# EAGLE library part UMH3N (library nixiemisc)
UMT6
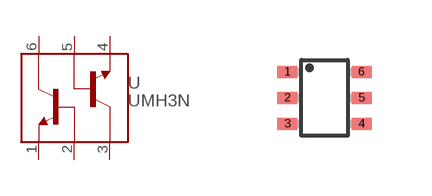
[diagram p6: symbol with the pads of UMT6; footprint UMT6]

Designator prefix U

## UMH3NUMT6  [UMT6]
1  E1  out
2  B1  in
3  C2  in
4  E2  out
5  B2  in
6  C1  in

## Footprint UMT6 (pad centres in mm)
UMT6 Package EIAJ: SC-88 Source: http://www.rohm.com/products/databook/tr/pdf/umx1n.pdf
smd 0.5 x 0.3: 1 -0.925,0.65; 2 -0.925,0; 3 -0.925,-0.65; 4 0.925,-0.65; 5 0.925,0; 6 0.925,0.65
